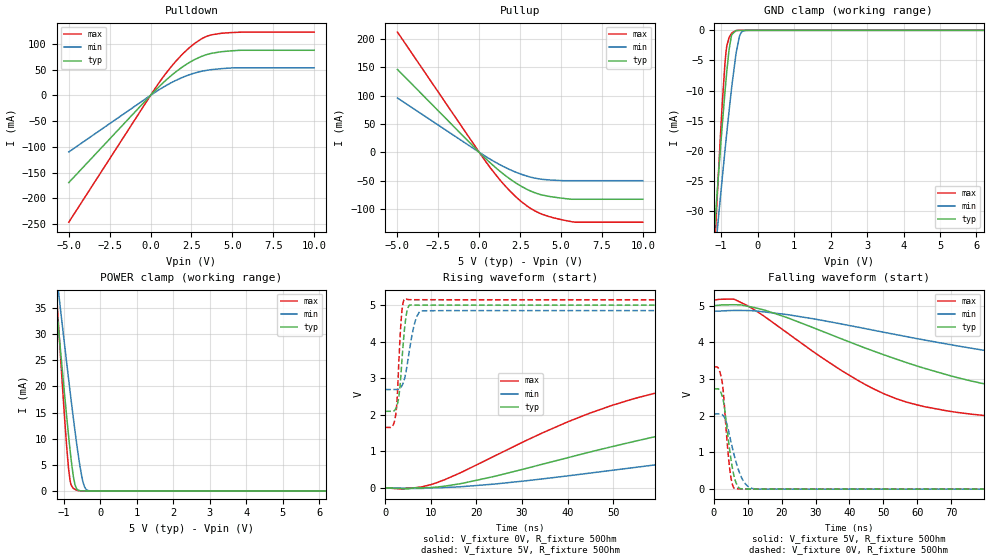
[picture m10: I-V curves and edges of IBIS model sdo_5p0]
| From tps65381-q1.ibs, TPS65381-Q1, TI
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|   sdo_5p0 Model
[Model]   sdo_5p0
Model_type   I/O
Polarity   Non-Inverting
Enable   Active-High
Vinl = 1.5
Vinh = 3.5
Vmeas = 2.5
Vref = 0
Cref = 100pF
Rref = 100
|   typ   min   max
|   (nom PVT)   (fast PVT)   (slow PVT)
C_comp   1.530e-12   1.500e-12   1.599e-12
[Model spec]
|subparameter
Vinl   1.5   1.455   1.545
Vinh   3.5   3.395   3.605
| Where nom  PVT is Nominal Process, 5V, 27C
|   Fast PVT is Strong Process,  5.15V, -40C
|   Slow PVT is Weak Process,   4.85V, 150C
[Voltage Range]   5   4.85   5.15
|Junction Temperature
[Temperature Range]   27   150   -40
[Pullup Reference]   5   4.85   5.15
[Pulldown Reference]   0   0   0
[Power Clamp Reference]   5   4.85   5.15
[GND Clamp Reference]   0   0   0
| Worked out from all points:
|   slope of the pulldown table from 0 to 0.75 V, typ, clamps not added: 31.4 ohm
|   slope of the pullup table from 0 to 0.75 V, typ, clamps not added: 36.4 ohm
|   GND clamp passes 1 mA (typ) near -0.72 V on its own axis
|   POWER clamp passes 1 mA (typ) near -0.68 V on its own axis
|   falling waveform, V_fixture 5V, R_fixture 50Ohm: 20-80 % time 63.5ns typ, 102ns min, 38.9ns max; typ from 5 V to 2.09 V
|   rising waveform, V_fixture 0V, R_fixture 50Ohm: 20-80 % time 66.3ns typ, 105ns min, 41.6ns max; typ from 0 V to 2.73 V
|   rising waveform, V_fixture 5V, R_fixture 50Ohm: 20-80 % time 1.14ns typ, 1.81ns min, 847ps max; typ from 2.09 V to 5 V
|   falling waveform, V_fixture 0V, R_fixture 50Ohm: 20-80 % time 2.33ns typ, 3.52ns min, 1.77ns max; typ from 2.73 V to 0 V
[Pulldown]
|   Voltage   I(typ)   I(min)   I(max)
-5V       -169.2mA   -109.7mA   -246mA
455mV     14.85mA    9.582mA    21.58mA
1.175V    35.97mA    22.99mA    52.21mA
1.551V    45.74mA    29.08mA    66.35mA
2.008V    56.34mA    35.57mA    81.72mA
2.632V    68.34mA    42.67mA    99.14mA
3.091V    75.17mA    46.5mA     109.1mA
3.441V    79.13mA    48.6mA     114.6mA
4.291V    84.45mA    51.63mA    120.2mA
5.585V    87.4mA     53.44mA    122.5mA
10V       87.4mA     53.44mA    122.6mA
[GND Clamp]
|   Voltage   I(typ)   I(min)   I(max)
-5V       -422.8mA   -335.7mA   -584.1mA
-1.227V   -36.87mA   -41.09mA   -42.12mA
-1.086V   -25.03mA   -31.92mA   -25.13mA
-972.7mV  -15.98mA   -24.75mA   -12.51mA
-895.4mV  -10.24mA   -20mA      -5.459mA
-864.6mV  -8.105mA   -18.15mA   -3.494mA
-785mV    -3.345mA   -13.52mA   -1.243mA
-720mV    -961.1uA   -9.941mA   -543.5uA
-591.4mV  -38.76uA   -3.816mA   -37.07uA
-474.9mV  -1.514uA   -646.7uA   -975.1nA
-305.2mV  0A         -14.4uA    0A
10V       0A         0A         0A
[Pullup]
|   Voltage   I(typ)   I(min)   I(max)
-5V       146.2mA    95.86mA    212.2mA
407.5mV   -11.49mA   -7.588mA   -16.78mA
1.51V     -39.12mA   -25.58mA   -56.87mA
1.895V    -47.42mA   -30.88mA   -68.85mA
2.58V     -60.15mA   -38.85mA   -87.17mA
3.178V    -68.84mA   -44.07mA   -99.68mA
3.832V    -75.29mA   -47.63mA   -109.2mA
4.502V    -78.85mA   -49.16mA   -115.2mA
5.709V    -82.85mA   -50.11mA   -122.7mA
10V       -82.85mA   -50.11mA   -123.3mA
[POWER Clamp]
|   Voltage   I(typ)   I(min)   I(max)
-5V       346mA      284.8mA    486.2mA
-1.246V   38.9mA     44.24mA    42.95mA
-1.1V     27.56mA    35.28mA    26.73mA
-988.1mV  19.08mA    28.49mA    14.87mA
-869.7mV  10.57mA    21.44mA    4.262mA
-797.6mV  5.905mA    17.26mA    1.112mA
-735.8mV  2.653mA    13.77mA    481.1uA
-655mV    455.1uA    9.411mA    163.3uA
-557.4mV  40.05uA    4.713mA    18.8uA
-475mV    4.792uA    1.744mA    1.44uA
-319.7mV  51.64nA    52.9uA     0A
10V       0A         0A         0A
[Ramp]
R_load = 50
|   typ   min   max
dV/dt_r   1.63999/6.61691e-08   1.22891/1.04346e-07   1.99811/4.13176e-08
dV/dt_f   1.74417/6.35082e-08   1.29575/1.0222e-07   2.09849/3.88255e-08
[Falling Waveform]
V_fixture = 5V
V_fixture_min = 4.85V
V_fixture_max = 5.15V
R_fixture = 50Ohm
|   Time   V(typ)   V(min)   V(max)
0s        5V         4.85V      5.15V
6.05ns    5.023V     4.867V     5.172V
9.825ns   4.983V     4.865V     5.001V
38.08ns   4.079V     4.491V     3.206V
53.68ns   3.546V     4.211V     2.468V
71.8ns    3.039V     3.903V     2.09V
99.1ns    2.597V     3.523V     1.878V
165.2ns   2.263V     3.017V     1.717V
255.6ns   2.145V     2.807V     1.667V
750ns     2.093V     2.69V      1.653V
[Rising Waveform]
V_fixture = 0V
V_fixture_min = 0V
V_fixture_max = 0V
R_fixture = 50Ohm
|   Time   V(typ)   V(min)   V(max)
0s        823.5pV    162.4nV    645.6pV
3.925ns   -22.96mV   -9.75mV    -36.96mV
11.28ns   20.01mV    1.78mV     139.1mV
40.25ns   830.4mV    330.1mV    1.816V
58.7ns    1.385V     619.4mV    2.573V
75.55ns   1.798V     871.3mV    2.903V
105.4ns   2.275V     1.25V      3.12V
171.8ns   2.583V     1.754V     3.27V
258.5ns   2.686V     1.944V     3.316V
750ns     2.733V     2.048V     3.33V
[Rising Waveform]
V_fixture = 5V
V_fixture_min = 4.85V
V_fixture_max = 5.15V
R_fixture = 50Ohm
|   Time   V(typ)   V(min)   V(max)
0s        2.093V     2.689V     1.653V
2.25ns    2.152V     2.69V      1.951V
2.625ns   2.269V     2.689V     2.442V
3ns       2.498V     2.7V       3.458V
3.6ns     3.354V     2.776V     4.744V
4.575ns   4.689V     3.185V     5.164V
5.25ns    4.988V     3.712V     5.149V
6.525ns   5V         4.536V     5.146V
8.4ns     4.997V     4.844V     5.146V
750ns     5V         4.85V      5.15V
[Falling Waveform]
V_fixture = 0V
V_fixture_min = 0V
V_fixture_max = 0V
R_fixture = 50Ohm
|   Time   V(typ)   V(min)   V(max)
0s        2.733V     2.049V     3.33V
1.325ns   2.732V     2.049V     3.298V
2.45ns    2.535V     2.031V     2.915V
4.325ns   1.306V     1.593V     857.5mV
5.25ns    693.6mV    1.207V     212mV
6.375ns   214.3mV    791mV      17.22mV
7.575ns   22.29mV    445.4mV    5.896mV
9.95ns    3.396mV    82.66mV    2.01mV
12.47ns   1.3mV      2.812mV    2.58mV
750ns     37.69nV    395.6nV    3.836nV
